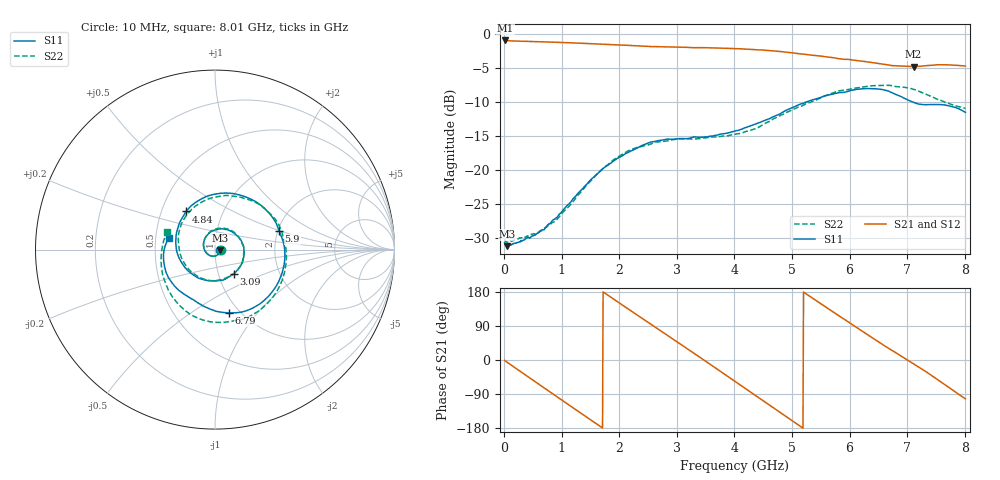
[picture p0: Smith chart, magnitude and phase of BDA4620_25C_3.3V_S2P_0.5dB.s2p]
!Agilent Technologies,E5071B,MY42404982,A.09.10
!Date: Wed May 06 08:56:03 2026
!Data & Calibration Information:
!Freq	S11:SOLT2(ON)	S21:SOLT2(ON)	S12:SOLT2(ON)	S22:SOLT2(ON)
# Hz S RI R 50
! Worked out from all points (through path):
!   801 points, 10 MHz to 8.01 GHz, reference 50 ohm
!   highest |S21| = -0.95 dB at 20 MHz (marker M1); lowest = -4.8 dB at 7.11 GHz (marker M2)
!   group delay of S21, straight-line fit = 285 ps
!   lowest |S11| = -31.2 dB at 60 MHz (marker M3), VSWR 1.06, Z = 52.8 - j0.437 ohm
!   |S11| at or under -10 dB: start of sweep to 5.248 GHz; 7.096 GHz to end of sweep
!   |S22| runs from -30.7 to -7.5 dB; largest |S21 - S12| = 0.0036
!   S11 on the Smith chart (normalised r, x): 10 MHz: 1.06, -0.00; 3.09 GHz: 1.18, -0.33; 4.84 GHz: 0.67, +0.31; 5.9 GHz: 2.03, +0.49; 6.79 GHz: 0.90, -0.73; 8.01 GHz: 0.59, +0.08
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1e7  0.0292 -0.00209  0.8957 -0.0193  0.897 -0.0193  0.0307 -0.00192
2e7  0.0282 -0.00269  0.8953 -0.0345  0.897 -0.0377  0.0304 -0.00128
6e7  0.0272 -0.00413  0.8863 -0.1027  0.8878 -0.1041  0.0291 -0.00324
7.3e8  -0.00938 -0.0369  0.1942 -0.8522  0.1939 -0.853  -0.00564 -0.0376
1.03e9  -0.0471 -0.0197  -0.2752 -0.82  -0.2759 -0.8209  -0.044 -0.0223
1.35e9  -0.064 0.0332  -0.6733 -0.5264  -0.6736 -0.527  -0.0638 0.0292
1.93e9  0.0281 0.1155  -0.7715 0.3127  -0.7721 0.3135  0.0223 0.1189
2.32e9  0.1233 0.0774  -0.3791 0.7241  -0.3807 0.7251  0.1205 0.0839
2.68e9  0.1631 -0.0229  0.1256 0.7963  0.1268 0.7971  0.161 -0.00728
3.09e9  0.104 -0.1346  0.6211 0.5038  0.6225 0.5031  0.1209 -0.119
3.54e9  -0.0265 -0.1739  0.784 -0.102  0.785 -0.1034  -0.00542 -0.173
4.01e9  -0.1617 -0.1054  0.4313 -0.6508  0.4313 -0.6522  -0.1488 -0.1068
4.42e9  -0.2184 0.0386  -0.124 -0.7542  -0.1259 -0.7541  -0.2037 0.0361
4.84e9  -0.1601 0.2128  -0.5945 -0.4396  -0.5952 -0.4398  -0.1364 0.2173
5.35e9  0.0964 0.3132  -0.6701 0.1933  -0.6709 0.1944  0.12 0.2951
5.9e9  0.3572 0.1049  -0.2053 0.6192  -0.2054 0.6187  0.3768 0.0828
6.26e9  0.3709 -0.1396  0.1942 0.5963  0.1961 0.5967  0.3805 -0.1509
6.68e9  0.1533 -0.3469  0.5089 0.2987  0.5102 0.2992  0.1918 -0.3729
6.79e9  0.0797 -0.3521  0.547 0.203  0.5489 0.2022  0.1154 -0.3949
7.11e9  -0.086 -0.3025  0.5667 -0.1005  0.568 -0.1018  -0.1072 -0.3771
7.62e9  -0.2634 -0.148  0.2831 -0.521  0.2835 -0.5233  -0.2936 -0.1272
8.01e9  -0.2568 0.067  -0.1259 -0.5672  -0.1264 -0.569  -0.2661 0.098
